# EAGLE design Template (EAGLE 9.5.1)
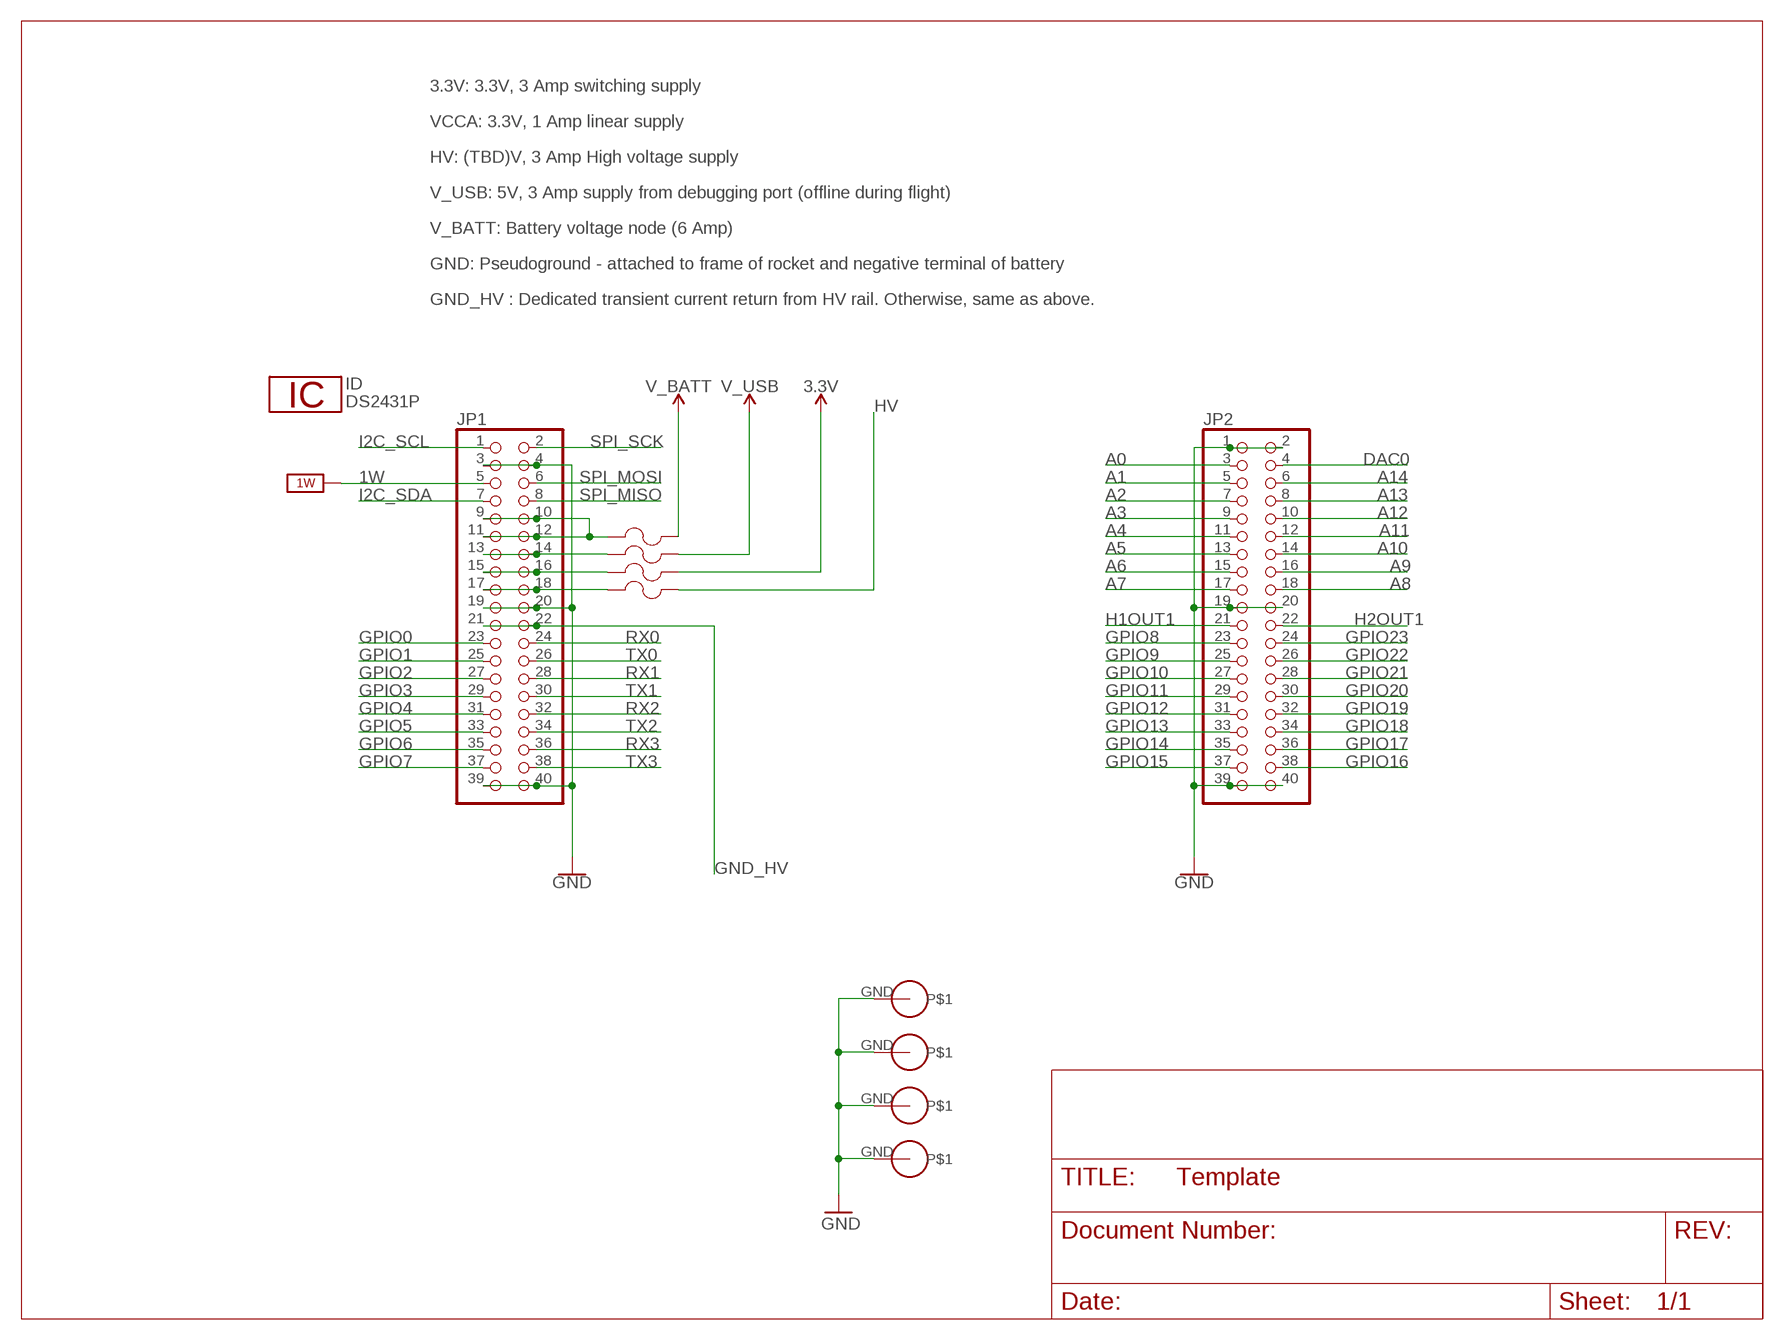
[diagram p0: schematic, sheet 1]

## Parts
F1  0603SFF150F/32-2  [FUS0603_TYCO]
F2  0603SFF150F/32-2  [FUS0603_TYCO]
F3  0603SFF150F/32-2  [FUS0603_TYCO]
F4  0603SFF150F/32-2  [FUS0603_TYCO]
ID  DS2431P  [TSOC6]
JP1  PINHD-2X20  [2X20]
JP2  PINHD-2X20  [2X20]
U$1  PS/104-MOUNTING-HOLE  [PC/104-MOUNTING-HOLE]
U$2  PS/104-MOUNTING-HOLE  [PC/104-MOUNTING-HOLE]
U$3  PS/104-MOUNTING-HOLE  [PC/104-MOUNTING-HOLE]
U$4  PS/104-MOUNTING-HOLE  [PC/104-MOUNTING-HOLE]

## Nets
1W: JP1.5 ; supply symbol labelled 1W_SUP
3.3V: F3.2
A0: JP2.3
A1: JP2.5
A2: JP2.7
A3: JP2.9
A4: JP2.11
A5: JP2.13
A6: JP2.15
A7: JP2.17
A8: JP2.18
A9: JP2.16
A10: JP2.14
A11: JP2.12
A12: JP2.10
A13: JP2.8
A14: JP2.6
DAC0: JP2.4
GND: JP1.3 JP1.4 JP1.19 JP1.20 JP1.39 JP1.40 JP2.1 JP2.2 JP2.19 JP2.20 JP2.39 JP2.40 U$1.GND U$2.GND U$3.GND U$4.GND
GND_HV: JP1.21 JP1.22
GPIO0: JP1.23
GPIO1: JP1.25
GPIO2: JP1.27
GPIO3: JP1.29
GPIO4: JP1.31
GPIO5: JP1.33
GPIO6: JP1.35
GPIO7: JP1.37
GPIO8: JP2.23
GPIO9: JP2.25
GPIO10: JP2.27
GPIO11: JP2.29
GPIO12: JP2.31
GPIO13: JP2.33
GPIO14: JP2.35
GPIO15: JP2.37
GPIO16: JP2.38
GPIO17: JP2.36
GPIO18: JP2.34
GPIO19: JP2.32
GPIO20: JP2.30
GPIO21: JP2.28
GPIO22: JP2.26
GPIO23: JP2.24
H1OUT1: JP2.21
H2OUT1: JP2.22
HV: F4.2
I2C_SCL: JP1.1
I2C_SDA: JP1.7
N$1: F4.1 JP1.17 JP1.18
N$2: F2.1 JP1.13 JP1.14
N$3: F3.1 JP1.15 JP1.16
N$4: F1.1 JP1.9 JP1.10 JP1.11 JP1.12
RX0: JP1.24
RX1: JP1.28
RX2: JP1.32
RX3: JP1.36
SPI_MISO: JP1.8
SPI_MOSI: JP1.6
SPI_SCK: JP1.2
TX0: JP1.26
TX1: JP1.30
TX2: JP1.34
TX3: JP1.38
V_BATT: F1.2
V_USB: F2.2

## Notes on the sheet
- 3.3V: 3.3V, 3 Amp switching supply
- VCCA: 3.3V, 1 Amp linear supply
- HV: (TBD)V, 3 Amp High voltage supply
- V_USB: 5V, 3 Amp supply from debugging port (offline during flight)
- V_BATT: Battery voltage node (6 Amp)
- GND: Pseudoground - attached to frame of rocket and negative terminal of battery
- GND_HV : Dedicated transient current return from HV rail. Otherwise, same as above.

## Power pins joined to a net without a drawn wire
1W: ID.2(1W)
GND: ID.1(GND)

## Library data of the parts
F1-F4 = CU inSpace 2019 Parts:0603SFF150F/32-2; MANUFACTURER_PART_NUMBER: 0603SFF150F322; VENDOR: Littelfuse Inc
ID = 1wire:DS2431: 1024-Bit EEPROM
JP1 JP2 = pinhead:PINHD-2X20: PIN HEADER
U$1-U$4 = CU inSpace 2019 Parts:PS/104-MOUNTING-HOLE: Mounting hole for PC/104 board.

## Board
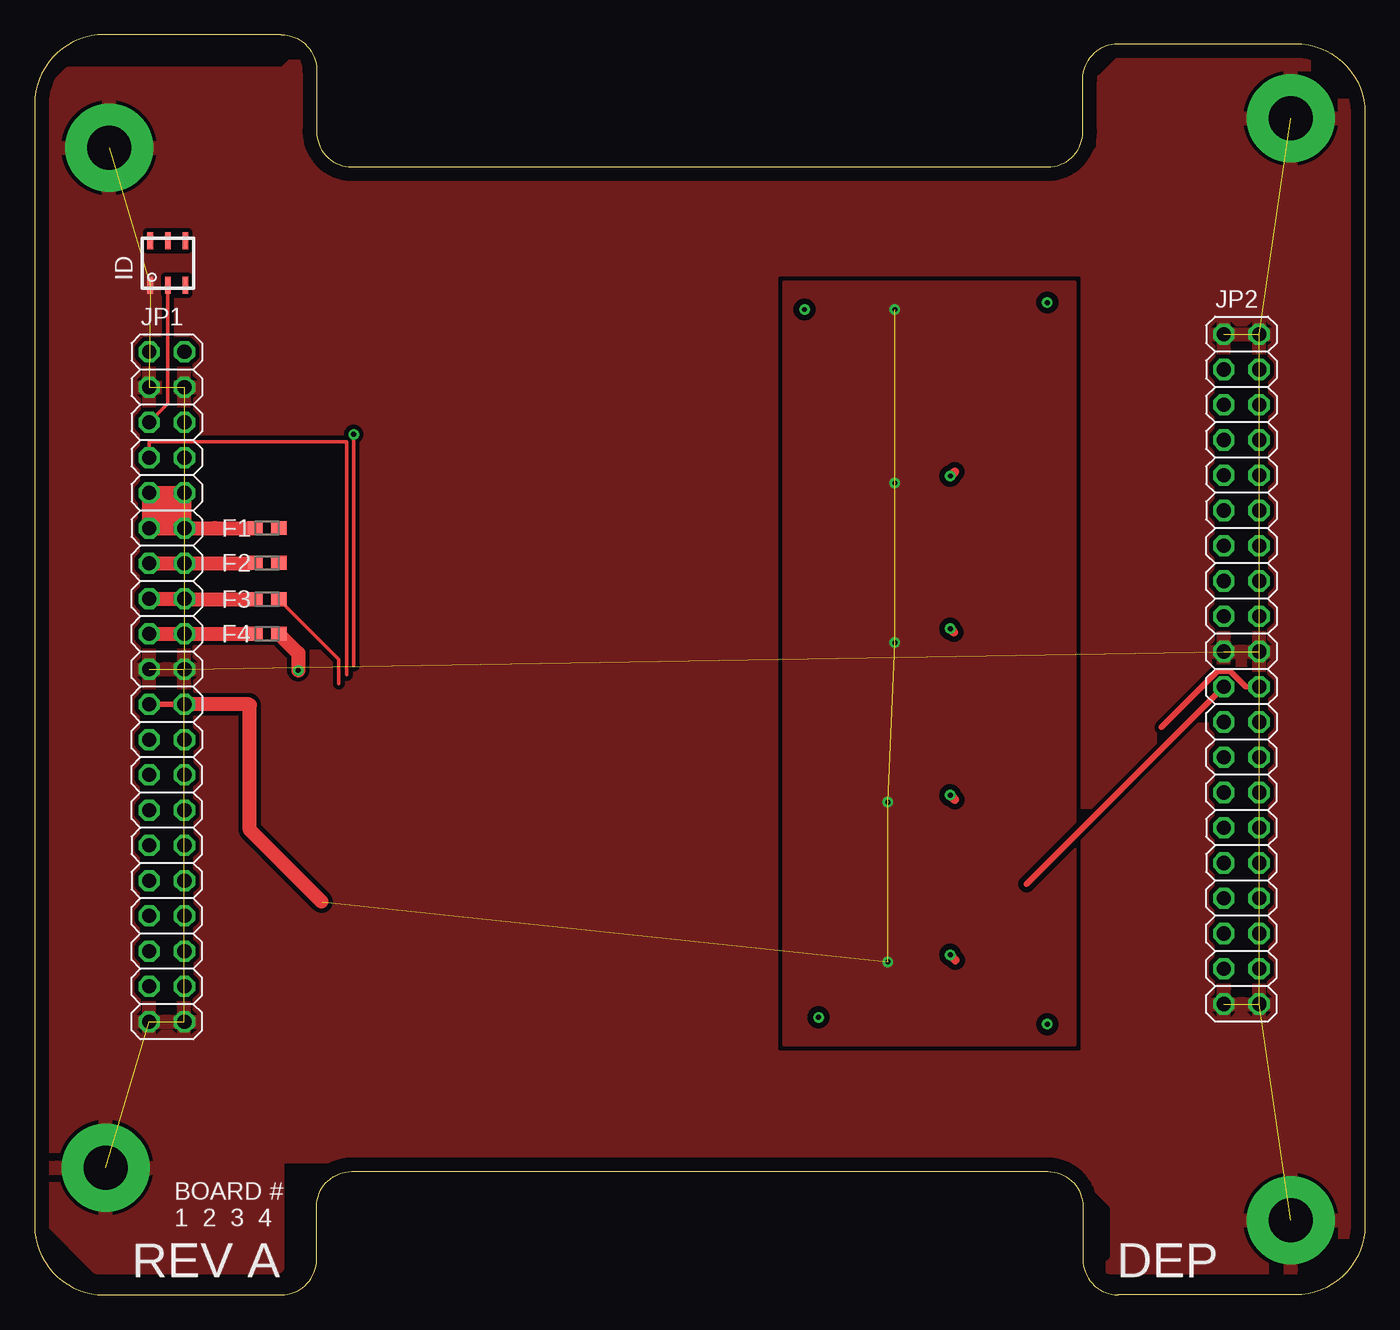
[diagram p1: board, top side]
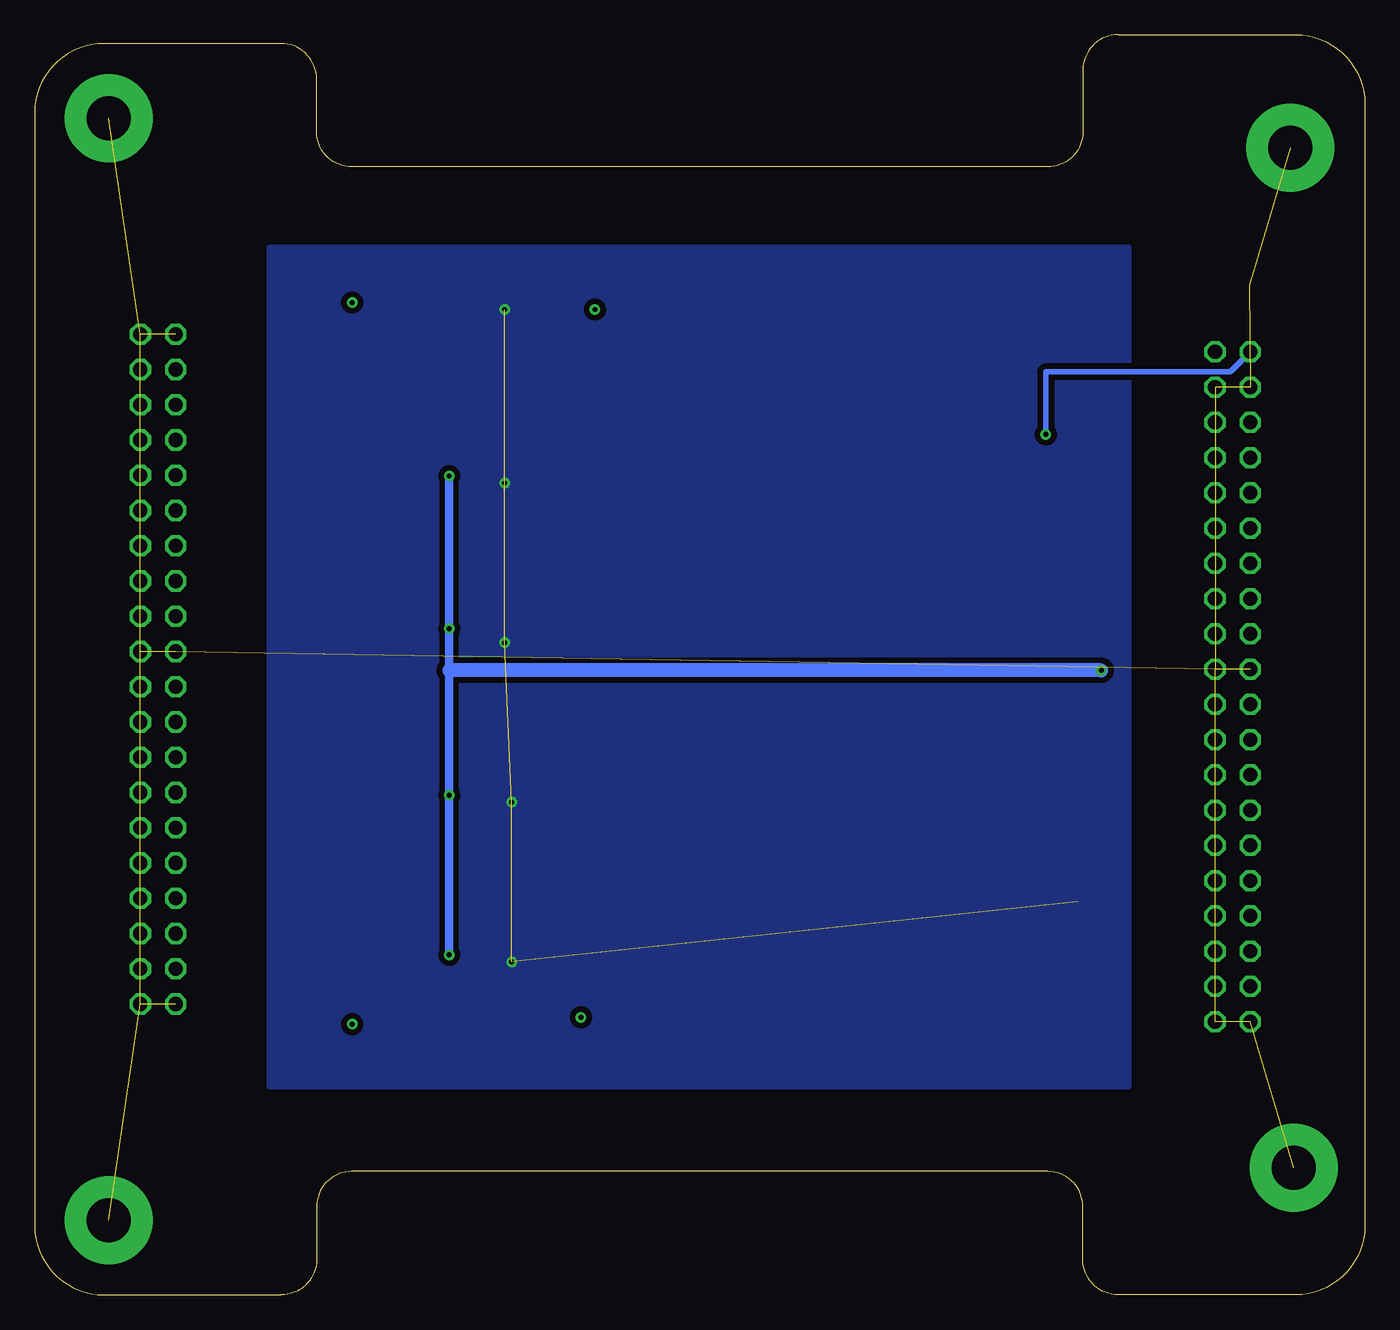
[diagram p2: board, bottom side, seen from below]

Size 95.89 x 90.81 mm. Coordinates in mm from the lower left corner, seen from the top.
Outline: 0,85.81 0,5 arc90 5,0 17.78,0 arc90 20.32,2.54 20.32,6.35 arc-90 22.86,8.89 73.03,8.89 arc-90 75.56,6.35 75.56,2.54 arc90 78.11,0 90.89,0 arc90 95.89,5 95.89,85.17 arc90 90.89,90.17 78.11,90.17 arc90 75.56,87.63 75.56,83.82 arc-90 73.03,81.28 22.86,81.28 arc-90 20.32,83.82 20.32,88.27 arc90 17.78,90.81 5,90.81 arc90 0,85.81
Copper layers (1*16): Top 0.035mm / dielectric 1.5mm / Bottom 0.035mm
Design rules "default": minimum track width 6mil, minimum drill 0.35mm, track to track 6mil, track to pad 6mil, pad to pad 6mil, via to via 6mil, smd to smd 6mil, copper to edge 40mil, drill to drill 6mil, minimum pad ring 10mil, minimum via ring 8mil, stop-mask expansion 4mil, vias tented up to drill 0mil, thermal gap 10mil

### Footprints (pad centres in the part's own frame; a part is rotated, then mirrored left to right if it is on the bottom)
FUS0603_TYCO = smd 1.092 x 0.991: 1 -0.851,0; 2 0.851,0
TSOC6 = smd 0.406 x 1.219: 1 -1.27,-1.6; 2 0,-1.6; 3 1.27,-1.6; 4 1.27,1.6; 5 0,1.6; 6 -1.27,1.6
2X20 = drill 1.016 octagon: 1 -24.13,-1.27; 2 -24.13,1.27; 3 -21.59,-1.27; 4 -21.59,1.27; 5 -19.05,-1.27; 6 -19.05,1.27; 7 -16.51,-1.27; 8 -16.51,1.27; 9 -13.97,-1.27; 10 -13.97,1.27; 11 -11.43,-1.27; 12 -11.43,1.27; 13 -8.89,-1.27; 14 -8.89,1.27; 15 -6.35,-1.27; 16 -6.35,1.27; 17 -3.81,-1.27; 18 -3.81,1.27; 19 -1.27,-1.27; 20 -1.27,1.27; 21 1.27,-1.27; 22 1.27,1.27; 23 3.81,-1.27; 24 3.81,1.27; 25 6.35,-1.27; 26 6.35,1.27; 27 8.89,-1.27; 28 8.89,1.27; 29 11.43,-1.27; 30 11.43,1.27; 31 13.97,-1.27; 32 13.97,1.27; 33 16.51,-1.27; 34 16.51,1.27; 35 19.05,-1.27; 36 19.05,1.27; 37 21.59,-1.27; 38 21.59,1.27; 39 24.13,-1.27; 40 24.13,1.27
PC/104-MOUNTING-HOLE = drill 3.175 pad 6.35: GND 0,0

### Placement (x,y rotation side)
F1  16.75,55.25 0 top
F2  16.75,52.75 0 top
F3  16.75,50.13 0 top
F4  16.75,47.63 0 top
ID  9.6,74.35 0 top
JP1  9.53,43.81 270 top
JP2  87,45.09 270 top
U$1  5.36,82.65 0 top
U$2  90.55,84.79 0 top
U$3  5.13,9.17 0 top
U$4  90.55,5.36 0 top

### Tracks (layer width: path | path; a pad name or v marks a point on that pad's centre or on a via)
1W
  Top 0.254: ID.2 9.6,64.21 JP1.5
3.3V
  Top 0.254: 21.93,44.04 21.93,45.8 F3.2
GND  (16 unrouted)
  pour Top (isolate 0.305, rank 2): 1,86 1,5.5 4.5,2 17.5,2 17.5,10 74.5,10 75,9.5 78,6.5 78,6 78,2.5 77.5,2 93.5,2 94.5,3 95,3 95,87 93,89 90.5,89 78.5,89 77,87.5 77,82.5 75,80.5 21,80.5 19,82.5 19,89 18,88 2.5,88 1,86.5
GND_HV  (via drill 0.35)  (5 unrouted)
  Top 0.406: JP1.21 JP1.22
  Top 1.016: JP1.22 15.46,42.55 15.5,42.5 15.5,33.5 20.68,28.32
  other vias: 62,71 62,58.5 62,47 61.5,35.5 61.5,24
  pour Top (isolate 0.406): 55,73 75,73 75,18 54,18 54,73
  pour Bottom (isolate 0.406): 17,75.5 79,75.5 79,15 17,15 17,75
H1OUT1
  Top 0.406: 71.5,29.59 JP2.21
H2OUT1
  Top 0.406: 81.22,40.9 85.26,44.93 86.19,44.93 87.31,43.81 JP2.22
HV  (via drill 0.35)
  Top 0.61: 66.25,47.75 v66,48 | 66.32,35.68 v66,36 | 66.39,24.11 v66,24.5 | 66.32,59.32 v66,59
  Top 1.016: F4.2 19,46.24 v19,45
  Bottom 0.61: v66,59 v66,48 66,45 v66,36 v66,24.5
  Bottom 1.016: v19,45 66,45
I2C_SCL  (via drill 0.35)
  Top 0.254: 23,45.34 v23,62
  Bottom 0.406: JP1.1 9.7,66.5 10.31,66.5 10.33,66.52 11.26,66.52 11.28,66.5 23,66.5 v23,62
I2C_SDA
  Top 0.254: 22.5,44.68 22.5,61.47 8.26,61.47 JP1.7
N$1
  Top 1.016: JP1.17 JP1.18 14.9,47.62 F4.1
N$2
  Top 1.016: JP1.13 JP1.14 14.9,52.7 F2.1
N$3
  Top 1.016: JP1.15 JP1.16 10.79,50.13 F3.1
N$4
  Top 1.016: 9,55.24 JP1.11 JP1.9 | 9,55.24 10,55.24 | 10,55.24 JP1.12 | JP1.12 13,55.24 14.9,55.24 F1.1 | JP1.9 10,57.78 | 10,57.78 JP1.10 JP1.12 | JP1.9 9,57.78 9,55.24 | 10,55.24 10,57.78
N$7  (via drill 0.35)
  other vias: 56.5,20
N$8  (via drill 0.35)
  other vias: 73,19.5
N$9  (via drill 0.35)
  other vias: 55.5,71
N$12  (via drill 0.35)
  other vias: 73,71.5

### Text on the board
tPlace: BOARD # / 1 2 3 4 | REV A | DEP
Notes: RF Connectors should go in this notch | Debug connectors should go in this notch | Indicator LEDs should be placed in the bottom corners, filling the avaliable space from left to right

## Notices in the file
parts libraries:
SparkFun-PowerSymbols: Licensing: Creative Commons ShareAlike 4.0 International - https://creativecommons.org/licenses/by-sa/4.0
